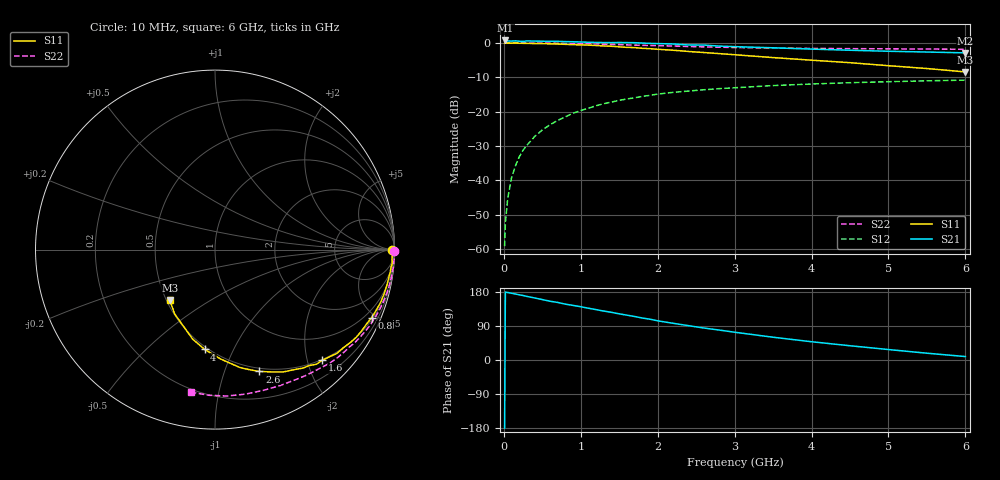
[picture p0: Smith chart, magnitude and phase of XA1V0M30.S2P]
! SIEMENS Discrete & RF Semiconductors
! BFY180
! Si NPN RF Bipolar Junction Transistor in MICRO-X
! VCE = 1 V  IC = 0.3 mA
! Common Emitter S-Parameters:  May  1997
# GHz  S  MA  R  50
!  f  S11  S21  S12  S22
! GHz  MAG  ANG  MAG  ANG  MAG  ANG  MAG  ANG
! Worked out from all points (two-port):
!   36 points, 10 MHz to 6 GHz, reference 50 ohm
!   highest |S21| = 0.69 dB at 20 MHz (marker M1); lowest = -2.9 dB at 6 GHz (marker M2)
!   |S21| within 3 dB of the highest: start of sweep to 4.754 GHz
!   lowest |S11| = -8.5 dB at 6 GHz (marker M3), VSWR 2.21, Z = 26.1 - j17.1 ohm
!   |S11| at or under -10 dB: nowhere
!   |S22| runs from -1.9 to 0.0 dB; largest |S21 - S12| = 1.1
!   S11 on the Smith chart (normalised r, x): 10 MHz: open; 800 MHz: 0.60, -4.74; 1.6 GHz: 0.49, -2.28; 2.6 GHz: 0.47, -1.32; 4 GHz: 0.48, -0.78; 6 GHz: 0.52, -0.34
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0.01  0.988 -0.1  1.044 -179.9  0.0011 98.1  0.9984 -0.3
0.02  0.9888 -0.5  1.083 179.1  0.0024 92.2  0.9999 -0.5
0.05  0.9883 -1.3  1.065 178.2  0.0054 90.2  0.9993 -1.1
0.1  0.9876 -3.1  1.061 176.2  0.0109 88.6  0.9985 -2.3
0.15  0.9905 -4.5  1.069 174.2  0.0161 86.4  0.9993 -3.3
0.2  0.9854 -5.8  1.056 172.0  0.0219 84.9  0.9979 -4.4
0.25  0.9845 -7.3  1.048 170.2  0.0274 84.6  0.9992 -5.6
0.3  0.981 -8.9  1.067 167.8  0.0324 82.9  0.9963 -6.6
0.4  0.978 -11.6  1.06 163.7  0.0433 80.2  0.9952 -8.7
0.6  0.9684 -17.7  1.053 155.1  0.0643 75.7  0.9896 -13.2
0.8  0.9511 -23.5  1.042 147.4  0.084 70.6  0.9816 -17.5
1.1  0.9262 -31.8  1.019 136.6  0.112 63.3  0.966 -23.8
1.6  0.8589 -45.8  1.008 118.3  0.1525 52.2  0.9351 -33.9
1.8  0.8323 -50.9  0.993 110.7  0.1661 48.3  0.9207 -37.6
2.2  0.7807 -60.8  0.963 96.9  0.1902 40.3  0.899 -44.8
2.6  0.7224 -70.0  0.928 84.4  0.2075 33.9  0.8737 -51.1
3  0.6713 -78.1  0.88 73.3  0.2218 27.6  0.8551 -57.3
3.5  0.6101 -87.1  0.847 60.1  0.2389 21.4  0.8403 -64.2
4  0.5593 -95.9  0.811 48.2  0.2518 15.1  0.829 -71.2
4.5  0.5141 -104.0  0.78 37.6  0.263 9.4  0.8227 -78.2
5.5  0.4228 -122.2  0.735 17.9  0.28 -1.5  0.8123 -92.5
6  0.3774 -131.8  0.715 9.1  0.2867 -7.2  0.8054 -99.6
